(* Logix 5000 AddOnInstructionDefinition export T2UU; software revision 32.02 *)

ADD_ON_INSTRUCTION T2UU   (* revision 1.0, vendor Exlar Corporation *)
// Help:
// Use the Tritex 2 User Units (T2UU) instruction to calculate user units. User units are easy-to-understand units of measurement that simplify your programming tasks. You define user units via parameters DistUUPerRev, VelTimeScale and CurrentScale.
// Configured for Exlar EIP AOI. 07/01/2014
// ----------------------------------------------------------------------------------------------------------------------------
// Parameters Bit Definition
// ----------------------------------------------------------------------------------------------------------------------------
// VelTimeScale:  (Input) Select the units you want for velocity.
//                          This will also effect acceleration
// ------------------------------------------------------------------
//      VelTimeScale = 0:     Seconds  (Velocity: Units/S,  Acceleration:  Units/S/S)
//      VelTimeScale = 1:     Minutes    (Velocity: Units/M, Acceleration:  Units/S/M)
// CurrentScale:  (Input) Select the units you want for Current
// ------------------------------------------------------------------
//      CurrentScale = 0:     AMPS
//      CurrentScale = 1:     % of Current Limit (Modbus ID 5108)
VAR_INPUT
   DistScale : REAL; {visible}   // Distance User Units Per Rev
   VelScale : REAL; {visible}   // Velocity Scale
   AccScale : REAL; {visible}   // Acceleration Scale
   CurrentScaling : INT; {visible}   // Current Scale
END_VAR
VAR_IN_OUT
   Units : REAL[5]; {required}   // Units Scale Results
        [0]   // Status
        [1]   // Distance
        [2]   // Velocity Scale
        [3]   // Acceleration Scale
        [4]   // Current Scaling Method
END_VAR
VAR_OUTPUT
   ER : BOOL; {access Read Only, visible}   // A Instruction error is Active
END_VAR

ROUTINE Logic   (* structured text *)
   (***********************************************)
   (*   Exlar Tritex 2 User Units                 *)
   (*                                             *)
   (***********************************************)
   
   
   
   (* Check for Error *)
   	if ((DistScale = 0) or (VelScale = 0)or (AccScale = 0 ))then
   		ER := 1;
   		Units[0] := 0;
   	else
   		ER := 0;
   		Units[0] := 1;
   	End_if;
   
   (* Load Global Units       *)
   	(* Current Scale       *)
   	(*       0: AMPs       *)
   	(*       1: % of Rated *)
   
   	(* Distance User Units per Rev *)
   	(*Units[0] := Units Status *)
   	Units[1] := DistScale;
   	Units[2] := VelScale;
   	Units[3] := AccScale;
   	Units[4] := CurrentScaling AND 16#1;
   
   
   
END_ROUTINE
END_ADD_ON_INSTRUCTION
